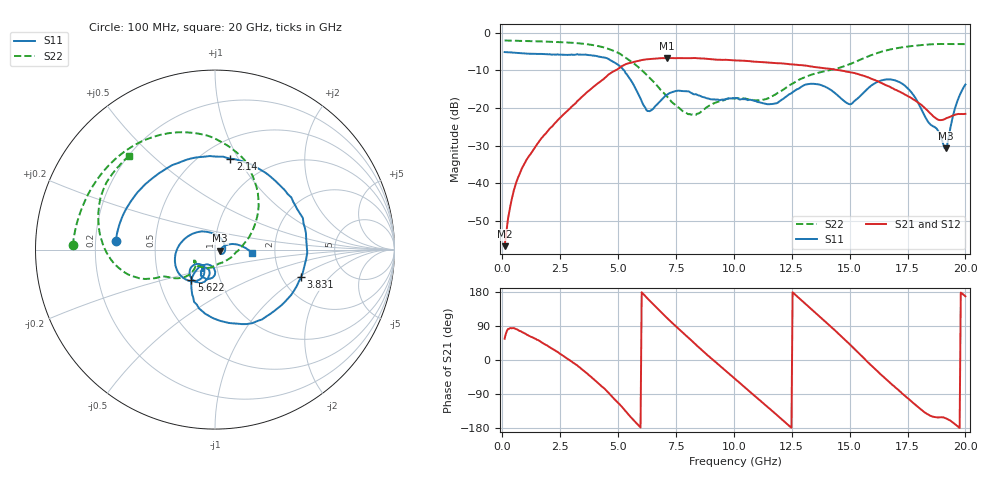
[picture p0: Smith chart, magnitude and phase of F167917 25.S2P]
!  2-Port S-parameters saved by WinCal
! VAR MeasName=S-Parameters (CALIBRATED_DATA) read from VNA (N5242A)
! VAR MeasDate=2016-11-22 9:00:57
! VAR NAME=F167917 25
! VAR FILENAME=F167917 25.S2P
! VAR DATE=2016-11-22 9:00:57
! VAR PHYS_PORTS=1,2
# Hz S DB R 50
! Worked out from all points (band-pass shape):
!   401 points, 100 MHz to 20 GHz, reference 50 ohm
!   highest |S21| = -6.69 dB at 7.115 GHz (marker M1); lowest = -56.7 dB at 100 MHz (marker M2)
!   |S21| within 3 dB of the highest: 4.974 GHz to 14.3 GHz (9.324 GHz wide, 96.8 % of centre)
!   lowest |S11| = -30.7 dB at 19.15 GHz (marker M3), VSWR 1.06, Z = 52.9 - j0.565 ohm
!   |S11| at or under -10 dB: 5.261 GHz to end of sweep
!   |S22| runs from -21.8 to -2.0 dB; largest |S21 - S12| = 0.0043
!   S11 on the Smith chart (normalised r, x): 100 MHz: 0.29, +0.04; 2.14 GHz: 0.67, +0.93; 3.831 GHz: 2.53, -1.05; 5.622 GHz: 0.73, -0.26; 20 GHz: 1.51, -0.06
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1e8  -5.12 175.3  -56.74 56.1  -57.07 55.4  -2.02 178.3
3.985e8  -5.22 161.5  -44.51 83.9  -44.41 84.5  -2.07 173.5
7.4675e8  -5.39 146.0  -37.57 76.7  -37.44 76.7  -2.13 168.2
2.13975e9  -5.79 80.3  -24.97 30.2  -24.97 30.0  -2.38 145.9
3.43325e9  -5.82 7.2  -17.06 -24.3  -17.07 -24.2  -2.86 120.2
3.83125e9  -5.95 -17.8  -14.90 -44.4  -14.89 -44.3  -3.17 110.5
4.62725e9  -7.11 -70.3  -10.91 -89.1  -10.89 -89.1  -4.38 87.3
5.62225e9  -13.32 -127.5  -7.84 -155.5  -7.80 -155.7  -7.85 54.3
6.269e9  -20.80 -115.1  -7.02 162.5  -7.01 162.3  -11.40 33.3
6.7665e9  -18.54 -90.1  -6.75 131.8  -6.75 131.8  -14.65 16.5
7.11475e9  -16.45 -93.2  -6.69 111.0  -6.70 111.0  -16.93 3.2
8.657e9  -17.06 -122.9  -6.82 24.1  -6.81 24.0  -20.65 -93.8
1.005e10  -17.44 -120.9  -7.32 -49.8  -7.32 -49.7  -17.42 -145.4
1.099525e10  -18.30 -123.5  -7.71 -99.7  -7.67 -99.7  -17.94 -149.7
1.204e10  -17.89 -104.0  -8.11 -154.8  -8.07 -154.7  -15.49 -136.0
1.338325e10  -13.56 -122.8  -8.96 132.2  -8.93 132.5  -11.06 -145.3
1.427875e10  -15.58 -143.3  -9.67 83.1  -9.66 83.3  -9.73 -152.7
1.5224e10  -18.05 -118.4  -10.71 28.1  -10.69 28.2  -7.78 -156.5
1.67165e10  -12.37 -150.3  -14.28 -58.4  -14.27 -58.3  -4.47 -177.2
1.7612e10  -15.41 154.8  -17.16 -106.1  -17.06 -106.2  -3.56 167.8
1.915425e10  -30.71 -10.5  -22.78 -153.9  -22.69 -153.5  -2.96 143.4
2e10  -13.75 -5.2  -21.55 167.9  -21.43 168.3  -3.00 132.5
